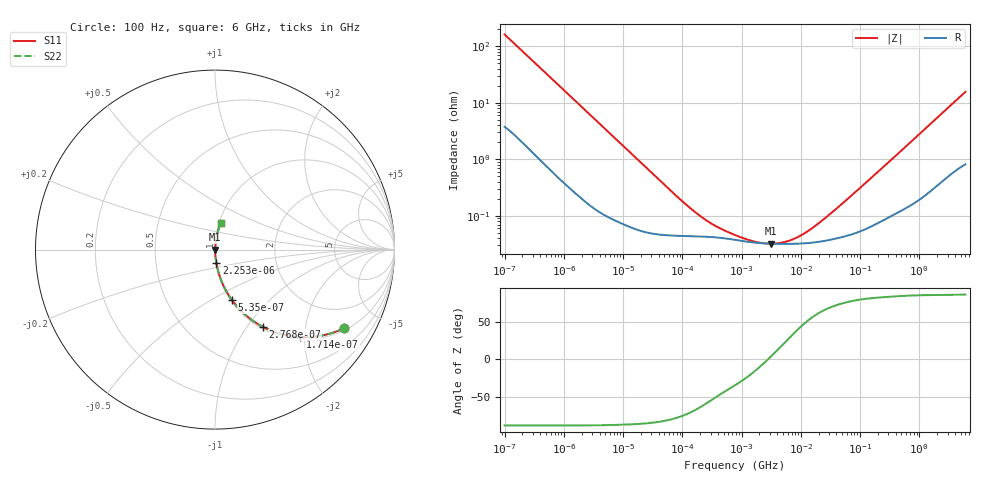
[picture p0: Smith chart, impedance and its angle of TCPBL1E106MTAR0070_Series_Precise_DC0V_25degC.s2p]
! TCPBL1E106MTAR0070 Polymer Tantalum Capacitor Sparameter Model
! Model Generated by Samsung Electro-Mechanics
! Samsung Sparameter Version 5.0
! Date : Oct-21-2025
! Products : Polymer Tantalum Capacitor
! Characteristics :
!  Nominal Capacitance = 10uF
!  Capacitance Tolerance = +/-20%
!  ESR = 70 mohm max at 100kHz
!  Rated Voltage = 25Vdc
!  Size = 1411(unit:inch), 3528(unit:mm)
!  Length = 3.50+/-0.20mm
!  Width = 2.80+/-0.20mm
!  Thickness = 1.10+/-0.10mm
!  Lineup = Conductive Polymer Type
!  Feature = PBL
!  Measurement Temperature : 25degC.
!  DC bias Value = 0V
!  Frequency : 100Hz ~ 6GHz
! External Node Assignments :
!  1  o---||---o  2
# MHz S RI R 50.0
! Freq.  Real(S11)  Im(S11)  Real(S12)  Im(S12)  Real(S21)  Im(S21)  Real(S22)  Im(S22)
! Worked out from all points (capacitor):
!   300 points, 100 Hz to 6 GHz, reference 50 ohm
!   read as one part in series: C = 9.8 uF near 106.2 Hz
!   lowest |Z| = 32.2 mohm at 3.165 MHz (marker M1)
!   series resonance near 2.786 MHz, so ESL is about 330 pH
!   S11 on the Smith chart (normalised r, x): 100 Hz: 1.08, -3.23; 171.4 Hz: 1.05, -1.90; 276.8 Hz: 1.03, -1.19; 535 Hz: 1.01, -0.62; 2.253 kHz: 1.00, -0.15; 6 GHz: 1.02, +0.31
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0.0001  0.7184 -0.4383  0.2816 0.4383  0.2816 0.4383  0.7184 -0.4383
0.0001714451  0.476 -0.4874  0.524 0.4874  0.524 0.4874  0.476 -0.4874
0.0002768446  0.2659 -0.4301  0.7341 0.4301  0.7341 0.4301  0.2659 -0.4301
0.0003735128  0.1694 -0.3637  0.8306 0.3637  0.8306 0.3637  0.1694 -0.3637
0.0005350431  0.0932 -0.2795  0.9068 0.2795  0.9068 0.2795  0.0932 -0.2795
0.00103405  0.029 -0.1567  0.971 0.1567  0.971 0.1567  0.029 -0.1567
0.001998454  0.00906 -0.0836  0.9909 0.0836  0.9909 0.0836  0.00906 -0.0836
0.002252796  0.00738 -0.0744  0.9926 0.0744  0.9926 0.0744  0.00738 -0.0744
0.007030492  0.00143 -0.0243  0.9986 0.0243  0.9986 0.0243  0.00143 -0.0243
0.03993819  0.000486 -0.00436  0.9995 0.00436  0.9995 0.00436  0.000486 -0.00436
0.1105667  0.000442 -0.00159  0.9996 0.00159  0.9996 0.00159  0.000442 -0.00159
0.2136865  0.000431 -0.000839  0.9996 0.000839  0.9996 0.000839  0.000431 -0.000839
0.3889699  0.000413 -0.000484  0.9996 0.000484  0.9996 0.000484  0.000413 -0.000484
0.7981464  0.000374 -0.000253  0.9996 0.000253  0.9996 0.000253  0.000374 -0.000253
1.738854  0.000334 -8.75e-05  0.9997 8.75e-05  0.9997 8.75e-05  0.000334 -8.75e-05
3.165205  0.000321 2.38e-05  0.9997 -2.38e-05  0.9997 -2.38e-05  0.000321 2.38e-05
6.895764  0.000319 0.000195  0.9997 -0.000195  0.9997 -0.000195  0.000319 0.000195
15.95059  0.000336 0.000518  0.9997 -0.000518  0.9997 -0.000518  0.000336 0.000518
46.88422  0.000417 0.00149  0.9996 -0.00149  0.9996 -0.00149  0.000417 0.00149
318.7652  0.00104 0.00924  0.999 -0.00924  0.999 -0.00924  0.00104 0.00924
1810.813  0.00553 0.0489  0.9945 -0.0489  0.9945 -0.0489  0.00553 0.0489
6000  0.0312 0.1496  0.9688 -0.1496  0.9688 -0.1496  0.0312 0.1496
